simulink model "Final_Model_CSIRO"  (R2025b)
settings: Solver=ode23tb  StartTime=0.0  StopTime=50  RelTol=1e-3
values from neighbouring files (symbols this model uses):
  C_4 = 0.1670*C_b    (= 1.00487241952e-06)    [VSM_CSIRO.m]    (also in VSM.m)
  C_6 = 0.2835*C_b    (= 1.70587623314e-06)    [VSM_CSIRO.m]    (also in VSM.m)
  C_8 = 0.2275*C_b    (= 1.36891302659e-06)    [VSM_CSIRO.m]    (also in VSM.m)
  C_dc = 0.008*(n)    (= 1.6)    [VSM_CSIRO.m]    (also in VSM.m)
  C_f = n*300*10^-6    (= 0.06)    [VSM_CSIRO.m]    (also in VSM.m)
  D_p = (1/(m_p*w_b))    (= 101321.183642)    [VSM_CSIRO.m]    (also in VSM.m)
  droop_percentage = 1    [VSM_CSIRO.m]    (also in VSM.m = 5)
  i_ll = -1.15*(S_b/Vdc_n)-i_loss_dc    [VSM_CSIRO.m]    (also in VSM.m)
  i_ul = 1.15*(S_b/Vdc_n)+i_loss_dc    [VSM_CSIRO.m]    (also in VSM.m)
  J = D_p*tau_f    (= 2026.42367285)    [VSM_CSIRO.m]    (also in VSM.m)
  k_dc = eta_1/(Vdc_n*m_p)    [VSM_CSIRO.m]    (also in VSM.m)
  K_p = (1/Vdc_n)    [VSM_CSIRO.m]    (also in VSM.m)
  K_r = 1/R_dc    [VSM_CSIRO.m]    (also in VSM.m)
  Kff_i = 1    [VSM_CSIRO.m]    (also in VSM.m)
  Kff_v = 1    [VSM_CSIRO.m]    (also in VSM.m)
  Ki_i = (1/n)*1.19    (= 0.00595)    [VSM_CSIRO.m]    (also in VSM.m)
  Ki_v = (n)*1.161022    (= 232.2044)    [VSM_CSIRO.m]    (also in VSM.m)
  ki_v_ac = 4*5.2500e-04    (= 0.0021)    [VSM_CSIRO.m]    (also in VSM.m)
  Kp_i = 0.738891    [VSM_CSIRO.m]    (also in VSM.m)
  Kp_v = 0.52    [VSM_CSIRO.m]    (also in VSM.m)
  kp_v_ac = 0.001    [VSM_CSIRO.m]    (also in VSM.m)
  L1_pu = 1*0.0186/m    (= 0.000186)    [VSM_CSIRO.m]    (also in VSM.m)
  L_45 = L_lines(2)    [VSM_CSIRO.m]    (also in VSM.m)
  L_56 = L_lines(3)    [VSM_CSIRO.m]    (also in VSM.m)
  L_67 = L_lines(5)    [VSM_CSIRO.m]    (also in VSM.m)
  L_78 = L_lines(6)    [VSM_CSIRO.m]    (also in VSM.m)
  L_89 = L_lines(8)    [VSM_CSIRO.m]    (also in VSM.m)
  L_94 = L_lines(9)    [VSM_CSIRO.m]    (also in VSM.m)
  L_f = (1/n)*200*10^-6    (= 1e-06)    [VSM_CSIRO.m]    (also in VSM.m)
  n = 200    [VSM_CSIRO.m]    (also in VSM.m)
  pl = S_b*ps    (= 75000000)    [VSM_CSIRO.m]    (also in VSM.m)
  ps = base/3    (= 0.75)    [VSM_CSIRO.m]    (also in VSM.m)
  R1_pu = 1*0.00734/m    (= 7.34e-05)    [VSM_CSIRO.m]    (also in VSM.m)
  R_45 = R_lines(2)    [VSM_CSIRO.m]    (also in VSM.m)
  R_56 = R_lines(3)    [VSM_CSIRO.m]    (also in VSM.m)
  R_67 = R_lines(5)    [VSM_CSIRO.m]    (also in VSM.m)
  R_78 = R_lines(6)    [VSM_CSIRO.m]    (also in VSM.m)
  R_89 = R_lines(8)    [VSM_CSIRO.m]    (also in VSM.m)
  R_94 = R_lines(9)    [VSM_CSIRO.m]    (also in VSM.m)
  R_dc = (Vdc_n/(0.05*(S_b)/Vdc_n))    [VSM_CSIRO.m]    (also in VSM.m)
  R_f = 0.001/n    (= 5e-06)    [VSM_CSIRO.m]    (also in VSM.m)
  S_b = 100*(10^6)    (= 100000000)    [VSM_CSIRO.m]    (also in VSM.m)
  S_bt = S_b    (= 100000000)    [VSM_CSIRO.m]    (also in VSM.m)
  T_en = T_load-0.5    (= 44.5)    [VSM_CSIRO.m]    (also in VSM.m = 24.5)
  t_l = 2    [VSM_CSIRO.m]
  tau_dc = 0.05    [VSM_CSIRO.m]    (also in VSM.m)
  tau_g = 5    [VSM_CSIRO.m]    (also in VSM.m)
  V1_rms = 1000    [VSM_CSIRO.m]    (also in VSM.m)
  V2_rms = 13800    [VSM_CSIRO.m]    (also in VSM.m)
  V_m = sqrt(2/3)*V1_rms    [VSM_CSIRO.m]    (also in VSM.m)
  Vdc_n = 3*V_m    [VSM_CSIRO.m]    (also in VSM.m)
  w_b = 2*pi*f_b    (= 314.159265359)    [VSM_CSIRO.m]    (also in VSM.m)
  w_f = 2*pi*5    (= 31.4159265359)    [VSM_CSIRO.m]    (also in VSM.m)
undefined symbols (not defined in the file or in its folder): D1, Delta, DiscIntNeverNeededParam, i_dc
libraries: spsSeriesRLCBranchLib x142, spsThreePhaseVIMeasurementLib x69, slpidlib x44, spsabctodq0Lib x44, spsVoltageMeasurementLib x28, spsGroundLib x23, spsThreePhaseBreakerLib x23, spsThreePhaseParallelRLCLoadLib x21, spsdq0toabcLib x16, spsUniversalBridgeLib x16, spsPowerPositiveSequenceLib x14, spsDCVoltageSourceLib x14
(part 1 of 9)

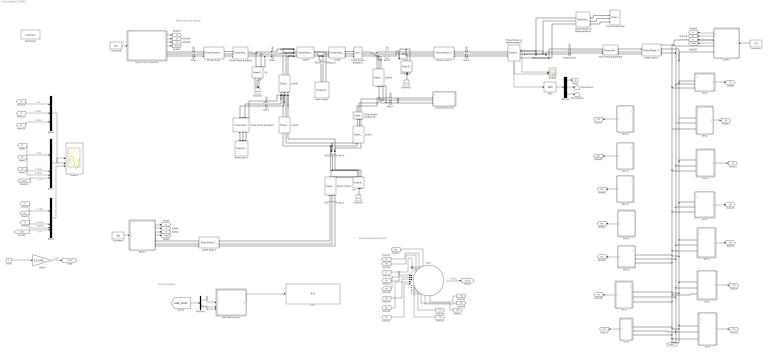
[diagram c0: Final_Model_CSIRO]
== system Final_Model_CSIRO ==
  note: Summation Block for GFLs
  note: IEEE 9-bus Test System
  note: SCR Calculation
  " " : spsThreePhaseVIMeasurementLib/Three-Phase V-I Measurement  VoltageMeasurement=no  SetLabelV=on  LabelV=Vabc_8  Vpu=on  VpuLL=off  CurrentMeasurement=no  SetLabelI=on  LabelI=Iabc_8  Ipu=on  Pbase=S_b  Vbase=V_b  OutputType=Complex  PhasorSimulation=off  PSBequivalent=0
  Base Load 5 : spsThreePhaseParallelRLCLoadLib/Three-Phase Parallel RLC Load  LConnTagsString=A|B|C  Configuration=Y (grounded)  NominalVoltage=230e3  Vabc=[1e3 1e3 1e3]  Vabcp=[1e3 1e3 1e3]  NominalFrequency=50  UnbalancedPower=off  ActivePower=pl  InductivePower=0  CapacitivePower=0  Pabc=[10e3 9e3 11e3]  QLabc=[100 90 110]  QCabc=[100 90 110]  Pabcp=[10e3 9e3 11e3]  QLabcp=[100 90 110]  QCabcp=[100 90 110]  Measurements=None  LoadType=constant Z
  "Base Load 9 " : spsThreePhaseParallelRLCLoadLib/Three-Phase Parallel RLC Load  LConnTagsString=A|B|C  Configuration=Y (grounded)  NominalVoltage=230e3  Vabc=[1e3 1e3 1e3]  Vabcp=[1e3 1e3 1e3]  NominalFrequency=50  UnbalancedPower=off  ActivePower=pl  InductivePower=0  CapacitivePower=0  Pabc=[10e3 9e3 11e3]  QLabc=[100 90 110]  QCabc=[100 90 110]  Pabcp=[10e3 9e3 11e3]  QLabcp=[100 90 110]  QCabcp=[100 90 110]  Measurements=None  LoadType=constant Z
  Bus 2 : spsThreePhaseVIMeasurementLib/Three-Phase V-I Measurement  VoltageMeasurement=no  SetLabelV=on  LabelV=Vabc_8  Vpu=on  VpuLL=off  CurrentMeasurement=no  SetLabelI=on  LabelI=Iabc_8  Ipu=on  Pbase=S_b  Vbase=V_b  OutputType=Complex  PhasorSimulation=off  PSBequivalent=0
  Bus 3 : spsThreePhaseVIMeasurementLib/Three-Phase V-I Measurement  VoltageMeasurement=no  SetLabelV=off  LabelV=Vabc_6  Vpu=off  VpuLL=off  CurrentMeasurement=no  SetLabelI=off  LabelI=Iabc_6  Ipu=off  Pbase=S_b  Vbase=V_b  OutputType=Complex  PhasorSimulation=off  PSBequivalent=0
  Bus 5 : spsThreePhaseVIMeasurementLib/Three-Phase V-I Measurement  VoltageMeasurement=no  SetLabelV=on  LabelV=Vabc_5  Vpu=on  VpuLL=off  CurrentMeasurement=no  SetLabelI=on  LabelI=Iabc_5  Ipu=on  Pbase=S_b  Vbase=V_b  OutputType=Complex  PhasorSimulation=off  PSBequivalent=0
  Bus 6 : spsThreePhaseVIMeasurementLib/Three-Phase V-I Measurement  VoltageMeasurement=no  SetLabelV=off  LabelV=Vabc_6  Vpu=off  VpuLL=off  CurrentMeasurement=no  SetLabelI=off  LabelI=Iabc_6  Ipu=off  Pbase=S_b  Vbase=V_b  OutputType=Complex  PhasorSimulation=off  PSBequivalent=0
  Bus 7 : spsThreePhaseVIMeasurementLib/Three-Phase V-I Measurement  VoltageMeasurement=no  SetLabelV=on  LabelV=Vabc_5  Vpu=on  VpuLL=off  CurrentMeasurement=no  SetLabelI=on  LabelI=Iabc_5  Ipu=on  Pbase=S_b  Vbase=V_b  OutputType=Complex  PhasorSimulation=off  PSBequivalent=0
  Bus 8 : spsThreePhaseVIMeasurementLib/Three-Phase V-I Measurement  VoltageMeasurement=no  SetLabelV=on  LabelV=Vabc_8  Vpu=on  VpuLL=off  CurrentMeasurement=no  SetLabelI=on  LabelI=Iabc_8  Ipu=on  Pbase=S_b  Vbase=V_b  OutputType=Complex  PhasorSimulation=off  PSBequivalent=0
  Bus 9 : spsThreePhaseVIMeasurementLib/Three-Phase V-I Measurement  VoltageMeasurement=no  SetLabelV=on  LabelV=Vabc_9  Vpu=on  VpuLL=off  CurrentMeasurement=no  SetLabelI=on  LabelI=Iabc_9  Ipu=on  Pbase=S_b  Vbase=V_b  OutputType=Complex  PhasorSimulation=off  PSBequivalent=0
  Bus1 : spsThreePhaseVIMeasurementLib/Three-Phase V-I Measurement  VoltageMeasurement=no  SetLabelV=on  LabelV=Vabc_1  Vpu=on  VpuLL=off  CurrentMeasurement=no  SetLabelI=on  LabelI=Iabc_1  Ipu=on  Pbase=S_b  Vbase=V_b  OutputType=Complex  PhasorSimulation=off  PSBequivalent=0
  Bus4 : spsThreePhaseVIMeasurementLib/Three-Phase V-I Measurement  VoltageMeasurement=no  SetLabelV=on  LabelV=Vabc_4  Vpu=on  VpuLL=off  CurrentMeasurement=no  SetLabelI=on  LabelI=Iabc_4  Ipu=on  Pbase=S_b  Vbase=V_b  OutputType=Complex  PhasorSimulation=off  PSBequivalent=0
  C4 : spsThreePhaseParallelRLCBranchLib/Three-Phase Parallel RLC Branch  LConnTagsString=A|B|C  RConnTagsString=A|B|C  BranchType=C  Resistance=1  Inductance=1e-3  Capacitance=C_4  Measurements=None
  C6 : spsThreePhaseParallelRLCBranchLib/Three-Phase Parallel RLC Branch  LConnTagsString=A|B|C  RConnTagsString=A|B|C  BranchType=C  Resistance=1  Inductance=1e-3  Capacitance=C_6  Measurements=None
  C8 : spsThreePhaseParallelRLCBranchLib/Three-Phase Parallel RLC Branch  LConnTagsString=A|B|C  RConnTagsString=A|B|C  BranchType=C  Resistance=1  Inductance=1e-3  Capacitance=C_8  Measurements=None
  Constant1 : Constant  Value=ps
  Constant3 : Constant  Value=0.1
  Constant8 : Constant  Value=ps
  Demux : Demux  Outputs=3
  Demux1 : Demux  Outputs=3
  Dummy Bus : spsThreePhaseVIMeasurementLib/Three-Phase V-I Measurement  VoltageMeasurement=no  SetLabelV=on  LabelV=Vabc_8  Vpu=on  VpuLL=off  CurrentMeasurement=no  SetLabelI=on  LabelI=Iabc_8  Ipu=on  Pbase=S_b  Vbase=V_b  OutputType=Complex  PhasorSimulation=off  PSBequivalent=0
  From : From
  GFL1 : Subsystem
  GFL10 : Subsystem
  GFL11 : Subsystem
  GFL12 : Subsystem
  GFL13 : Subsystem
  GFL14 : Subsystem
  GFL2 : Subsystem
  GFL3 : Subsystem
  GFL4 : Subsystem
  GFL5 : Subsystem
  GFL6 : Subsystem
  GFL7 : Subsystem
  GFL8 : Subsystem
  GFL9 : Subsystem
  GFM 1 : Subsystem
  GFM 2 : Subsystem
  Gain4 : Gain  Gain=1/(13.8e3)
  Goto7 : Goto
  Ground1 : spsGroundLib/Ground  LConnTagsString=a
  Ground2 : spsGroundLib/Ground  LConnTagsString=a
  Ground3 : spsGroundLib/Ground  LConnTagsString=a
  Incremental Load : Subsystem
  LV/MV Trafo 1 : spsThreePhaseTransformerTwoWindingsLib/Three-Phase Transformer (Two Windings)  Winding1Connection=Yg  Winding2Connection=Yg  CoreType=Three single-phase transformers  SetSaturation=off  Hysteresis=off  DataFile='hysteresis'  SetInitialFlux=off  Measurements=None  UNITS=pu  NominalPower=[S_bt 50 ]  Winding1="[ V1_rms R1_pu  L1_pu]"  Winding2=[ V2_rms R1_pu L1_pu]  Rm=Rm_pu  Lm=Lm_pu  L0=0.5  Saturation="[ 0,0  ;  0.005,1.2  ;  1.0,1.4 ]"  InitialFluxes=[ 0.8 , -0.8 , 0.7 ]  BreakLoop=off  DiscreteSolver=Trapezoidal iterative  DataType=off  TransfoNumber=0
  LV/MV Trafo 2 : spsThreePhaseTransformerTwoWindingsLib/Three-Phase Transformer (Two Windings)  Winding1Connection=Yg  Winding2Connection=Yg  CoreType=Three single-phase transformers  SetSaturation=off  Hysteresis=off  DataFile='hysteresis'  SetInitialFlux=off  Measurements=None  UNITS=pu  NominalPower=[ S_bt 50 ]  Winding1="[ V1_rms R1_pu  L1_pu]"  Winding2=[ V2_rms R1_pu L1_pu]  Rm=Rm_pu  Lm=Lm_pu  L0=0.5  Saturation="[ 0,0  ;  0.005,1.2  ;  1.0,1.4 ]"  InitialFluxes=[ 0.8 , -0.8 , 0.7 ]  BreakLoop=off  DiscreteSolver=Trapezoidal iterative  DataType=off  TransfoNumber=0
  Line45 : spsThreePhaseSeriesRLCBranchLib/Three-Phase Series RLC Branch  LConnTagsString=A|B|C  RConnTagsString=A|B|C  BranchType=RL  Resistance=R_45  Inductance=L_45  Capacitance=0  Measurements=None
  Line56 : spsThreePhaseSeriesRLCBranchLib/Three-Phase Series RLC Branch  LConnTagsString=A|B|C  RConnTagsString=A|B|C  BranchType=RL  Resistance=R_56  Inductance=L_56  Capacitance=0  Measurements=None
  Line67 : spsThreePhaseSeriesRLCBranchLib/Three-Phase Series RLC Branch  LConnTagsString=A|B|C  RConnTagsString=A|B|C  BranchType=RL  Resistance=R_67  Inductance=L_67  Capacitance=0  Measurements=None
  Line78 : spsThreePhaseSeriesRLCBranchLib/Three-Phase Series RLC Branch  LConnTagsString=A|B|C  RConnTagsString=A|B|C  BranchType=RL  Resistance=R_78  Inductance=L_78  Capacitance=0  Measurements=None
  Line89 : spsThreePhaseSeriesRLCBranchLib/Three-Phase Series RLC Branch  LConnTagsString=A|B|C  RConnTagsString=A|B|C  BranchType=RL  Resistance=R_89  Inductance=L_89  Capacitance=0  Measurements=None
  Line94 : spsThreePhaseSeriesRLCBranchLib/Three-Phase Series RLC Branch  LConnTagsString=A|B|C  RConnTagsString=A|B|C  BranchType=RL  Resistance=R_94  Inductance=L_94  Capacitance=0  Measurements=None
  MATLAB Function : MATLAB Function  TreatAsAtomicUnit=on
  "MV/HV Trafo " : spsThreePhaseTransformerTwoWindingsLib/Three-Phase Transformer (Two Windings)  Winding1Connection=Delta (D1)  Winding2Connection=Yg  CoreType=Three single-phase transformers  SetSaturation=off  Hysteresis=off  DataFile='hysteresis'  SetInitialFlux=off  Measurements=None  UNITS=pu  NominalPower=[ 210e6 50 ]  Winding1="[V2_rms 0.0027  0.08]"  Winding2=[230e3 0.0027 0.08]  Rm=500  Lm=500  L0=0.5  Saturation="[ 0,0  ;  0.005,1.2  ;  1.0,1.4 ]"  InitialFluxes=[ 0.8 , -0.8 , 0.7 ]  BreakLoop=off  DiscreteSolver=Trapezoidal iterative  DataType=off  TransfoNumber=0
  "MV/HV Trafo 1 " : spsThreePhaseTransformerTwoWindingsLib/Three-Phase Transformer (Two Windings)  Winding1Connection=Yg  Winding2Connection=Yg  CoreType=Three single-phase transformers  SetSaturation=off  Hysteresis=off  DataFile='hysteresis'  SetInitialFlux=off  Measurements=None  UNITS=pu  NominalPower=[ 210e6 50 ]  Winding1=[V2_rms 0.0027 0.08]  Winding2=[ 230e3 0.0027 0.08]  Rm=500  Lm=500  L0=0.5  Saturation="[ 0,0  ;  0.005,1.2  ;  1.0,1.4 ]"  InitialFluxes=[ 0.8 , -0.8 , 0.7 ]  BreakLoop=off  DiscreteSolver=Trapezoidal iterative  DataType=off  TransfoNumber=0
  "MV/HV Trafo 2 " : spsThreePhaseTransformerTwoWindingsLib/Three-Phase Transformer (Two Windings)  Winding1Connection=Yg  Winding2Connection=Yg  CoreType=Three single-phase transformers  SetSaturation=off  Hysteresis=off  DataFile='hysteresis'  SetInitialFlux=off  Measurements=None  UNITS=pu  NominalPower=[ 210e6 50 ]  Winding1=[V2_rms 0.0027 0.08]  Winding2=[230e3 0.0027 0.08]  Rm=500  Lm=500  L0=0.5  Saturation="[ 0,0  ;  0.005,1.2  ;  1.0,1.4 ]"  InitialFluxes=[ 0.8 , -0.8 , 0.7 ]  BreakLoop=off  DiscreteSolver=Trapezoidal iterative  DataType=off  TransfoNumber=0
  Mux1 : Mux
  Mux2 : Mux
  Mux6 : Mux  Inputs=3
  Power2 : Scope  NumInputPorts=3
  RMS : spsRMSLib/RMS  TrueRMS=on  Freq=50  RMSInit=120  Ts=0
  SCR : Display
  Scope1 : Scope  NumInputPorts=2
  Sum : Sum  Inputs=|++++++++++++++
  Synchronous Machine : Subsystem
  Terminator1 : Terminator
  Terminator2 : Terminator
  Three-Phase V-I Measurement1 : spsThreePhaseVIMeasurementLib/Three-Phase V-I Measurement  VoltageMeasurement=phase-to-phase  SetLabelV=off  LabelV=Vabc  Vpu=off  VpuLL=off  CurrentMeasurement=yes  SetLabelI=off  LabelI=Iabc  Ipu=off  Pbase=100e6  Vbase=500e3  OutputType=Complex  PhasorSimulation=off  PSBequivalent=0
  Three-Phase V-I Measurement3 : spsThreePhaseVIMeasurementLib/Three-Phase V-I Measurement  VoltageMeasurement=phase-to-phase  SetLabelV=on  LabelV=Vabc_Fault  Vpu=off  VpuLL=off  CurrentMeasurement=yes  SetLabelI=on  LabelI=Iabc_Fault  Ipu=off  Pbase=100e6  Vbase=500e3  OutputType=Complex  PhasorSimulation=off  PSBequivalent=0
  Three-Phase Breaker1 : spsThreePhaseBreakerLib/Three-Phase Breaker  InitialState=closed  SwitchA=on  SwitchB=on  SwitchC=on  SwitchTimes=50  External=off  BreakerResistance=1  SnubberResistance=1e6  SnubberCapacitance=inf  Measurements=None
  Three-Phase Breaker10 : spsThreePhaseBreakerLib/Three-Phase Breaker  InitialState=open  SwitchA=on  SwitchB=on  SwitchC=on  SwitchTimes=[0 0.5 40]  External=off  BreakerResistance=0.01  SnubberResistance=1e6  SnubberCapacitance=inf  Measurements=None
  Three-Phase Breaker5 : spsThreePhaseBreakerLib/Three-Phase Breaker  InitialState=open  SwitchA=on  SwitchB=on  SwitchC=on  SwitchTimes=1  External=off  BreakerResistance=0.01  SnubberResistance=1e6  SnubberCapacitance=inf  Measurements=None
  Three-Phase Breaker6 : spsThreePhaseBreakerLib/Three-Phase Breaker  InitialState=open  SwitchA=on  SwitchB=on  SwitchC=on  SwitchTimes=10  External=off  BreakerResistance=0.01  SnubberResistance=1e6  SnubberCapacitance=inf  Measurements=None
  Three-Phase Breaker9 : spsThreePhaseBreakerLib/Three-Phase Breaker  InitialState=open  SwitchA=on  SwitchB=on  SwitchC=on  SwitchTimes=[0 0.5 35]  External=off  BreakerResistance=0.01  SnubberResistance=1e6  SnubberCapacitance=inf  Measurements=None
  Three-Phase Fault : spsThreePhaseFaultLib/Three-Phase Fault  InitialStates=0  FaultA=on  FaultB=on  FaultC=on  GroundFault=on  SwitchTimes=[0.1 0.2]  External=off  SwitchStatus=NaN  FaultResistance=0.001  GroundResistance=0.01  SnubberResistance=1e6  SnubberCapacitance=inf  Measurements=Fault voltages and currents
  powergui2 : sps_lib/powergui  Priority=1  SimulationMode=Discrete  SampleTime=1e-4  frequency=50  Iterations=50  frequencyindice=0  Pbase=100e6  ErrMax=0.0001  UnitsV=kV  UnitsW=MW  buscounter=0  FunctionMessages=off  echomessages=off  EnableUseOfTLC=off  CurrentSourceSwitches=off  DisableSnubberDevices=off  DisableRonSwitches=off  DisableVfSwitches=off  DisplayEquations=off  AutomaticDiscreteSolvers=off  SolverType=Tustin/Backward Euler (TBE)  Interpol=off  ExternalGateDelay=off  methode=off  Ts=100  x0status=blocks  SPID=off  SwTol=0  HookPort=off  NonlinearTolerance=1e-4  nMaxIteration=100  ContinueOnMaxIteration=off  RestoreLinks=warning  ResistiveCurrentMeasurement=off  Frange=[0:2:500]  Ylog=off  Xlog=on  ShowGrid=off  save=off  variable=ZData  structure=0  ZoomFFT=off  StartTime=0.0  cycles=1  DisplayStyle=1  fundamental=60  FreqAxis=off  MaxFrequency=1000  frequencyindicesteady=1  RmsSteady=1  display=off
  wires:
  [f1] -> Mux6/1  "f_SM"
  GFM 1/2(V) -> [V2]
  GFM 2/2(V) -> [V3]
  GFM 2/1(f) -> [f3]
  [P3] -> Mux1/3  "P_GFM2"
  Constant1/1 -> GFM 2/1(Pset)
  [P2] -> Mux1/2  "P_GFM1"
  GFM 2/3(P) -> [P3]
  GFM 1/4(Theta) -> [Theta2]
  [V1] -> Mux2/1  "V_SM"
  Synchronous Machine/1(f) -> [f1]
  GFM 1/3(P) -> [P2]
  [f3] -> Mux6/3  "f_GFM2"
  [P1] -> Mux1/1  "P_SM"
  [V3] -> Mux2/3  "V_GFM2"
  Constant8/1 -> Synchronous Machine/1(Pset)
  Mux6/1 -> Power2/1
  GFM 1/1(f) -> [f2]
  [V2] -> Mux2/2  "V_GFM1"
  Mux1/1 -> Power2/2
  Synchronous Machine/3(P) -> [P1]
  Synchronous Machine/4(Theta) -> [Theta1]
  GFM 2/4(Theta) -> [Theta3]
  Synchronous Machine/2(V) -> [V1]
  Mux2/1 -> Power2/3
  [f2] -> Mux6/2  "f_GFM1"
  Three-Phase V-I Measurement1/2 -> Scope1/1
  Three-Phase V-I Measurement1/1 -> RMS/1, Scope1/2
  [V_PCC] -> Mux2/4  "V_PCC"
  [Iabc_Fault] -> Demux1/1
  Demux1/1 -> MATLAB Function/1(Ia)
  Demux1/3 -> MATLAB Function/3(Ic)
  MATLAB Function/1(SCR) -> SCR/1
  Demux1/2 -> MATLAB Function/2(Ib)
  RMS/1 -> Demux/1
  Demux/3 -> Terminator2/1
  Demux/2 -> Terminator1/1
  Demux/1 -> Goto7/1
  From/1 -> Gain4/1
  Gain4/1 -> [V_PCC]  "V_PCC"
  GFL1/1(Out1) -> [P5]
  GFL2/1(Out1) -> [P6]
  GFL3/1(Out1) -> [P7]
  GFL4/1(Out1) -> [P8]
  GFL5/1(Out1) -> [P9]
  GFL6/1(Out1) -> [P10]
  GFL7/1(Out1) -> [P11]
  [P15] -> Sum/1
  [P5] -> Sum/2
  [P6] -> Sum/3
  [P7] -> Sum/4
  [P8] -> Sum/5
  [P9] -> Sum/6
  [P10] -> Sum/7
  [P11] -> Sum/8
  Sum/1 -> [P_GFLs]  "P_GFLs"
  [P_GFLs] -> Mux1/4  "P_GFL"
  GFL8/1(Out1) -> [P12]
  [P12] -> Sum/9
  GFL10/1(Out1) -> [P13]
  [P13] -> Sum/10
  GFL9/1(Out1) -> [P14]
  [P14] -> Sum/11
  GFL11/1(Out1) -> [P15]
  GFL12/1(Out1) -> [P16]
  Constant3/1 -> GFM 1/1(Pset)
  GFL13/1(Out1) -> [P17]
  GFL14/1(Out1) -> [P18]
  [P16] -> Sum/12
  [P17] -> Sum/13
  [P18] -> Sum/14
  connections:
  Bus4/RConn2 -- Three-Phase Breaker1/RConn2 -- C4/LConn2
  "MV/HV Trafo 2 "/RConn3 -- C6/LConn3 -- Bus 6/RConn3
  Bus 8/LConn2 -- C8/LConn2 -- "MV/HV Trafo 1 "/RConn2
  C6/RConn2 -- Ground3/LConn1 -- C6/RConn1 -- C6/RConn3
  Bus 7/RConn2 -- Three-Phase Breaker10/LConn2 -- Line78/RConn2
  C4/LConn1 -- Bus4/RConn1 -- Three-Phase Breaker1/RConn1
  Line67/RConn1 -- Line56/RConn1 -- Bus 6/LConn1
  Line94/RConn3 -- Bus 9/RConn1 -- Line89/LConn3
  Bus 8/LConn3 -- C8/LConn3 -- "MV/HV Trafo 1 "/RConn3
  Bus 7/RConn3 -- Three-Phase Breaker10/LConn3 -- Line78/RConn3
  Line94/LConn1 -- Bus4/LConn1 -- Line45/LConn1
  Line45/RConn2 -- Line56/LConn2 -- Bus 5/LConn2
  Line94/LConn2 -- Bus4/LConn2 -- Line45/LConn2
  Line94/LConn3 -- Bus4/LConn3 -- Line45/LConn3
  C8/RConn2 -- C8/RConn3 -- C8/RConn1 -- Ground2/LConn1
  Line45/RConn1 -- Line56/LConn1 -- Bus 5/LConn1
  C6/LConn1 -- "MV/HV Trafo 2 "/RConn1 -- Bus 6/RConn1
  Line45/RConn3 -- Line56/LConn3 -- Bus 5/LConn3
  Bus 9/RConn2 -- Line94/RConn2 -- Line89/LConn2
  Ground1/LConn1 -- C4/RConn2 -- C4/RConn3 -- C4/RConn1
  Bus 7/RConn1 -- Three-Phase Breaker10/LConn1 -- Line78/RConn1
  Bus 6/LConn2 -- Line67/RConn2 -- Line56/RConn2
  Bus 6/LConn3 -- Line56/RConn3 -- Line67/RConn3
  Line94/RConn1 -- Bus 9/RConn3 -- Line89/LConn1
  Bus 8/LConn1 -- C8/LConn1 -- "MV/HV Trafo 1 "/RConn1
  C6/LConn2 -- "MV/HV Trafo 2 "/RConn2 -- Bus 6/RConn2
  Bus4/RConn3 -- Three-Phase Breaker1/RConn3 -- C4/LConn3
  Bus 2/RConn1 -- "MV/HV Trafo 1 "/LConn3
  Bus 2/RConn2 -- "MV/HV Trafo 1 "/LConn2
  GFM 2/RConn3 -- LV/MV Trafo 2/LConn3
  GFM 2/RConn2 -- LV/MV Trafo 2/LConn2
  GFM 2/RConn1 -- LV/MV Trafo 2/LConn1
  Bus1/LConn3 -- "MV/HV Trafo "/LConn3
  Bus 2/RConn3 -- "MV/HV Trafo 1 "/LConn1
  "Base Load 9 "/LConn1 -- Bus 9/LConn3
  "Base Load 9 "/LConn3 -- Bus 9/LConn1
  Bus1/LConn2 -- "MV/HV Trafo "/LConn2
  Bus 3/LConn1 -- "MV/HV Trafo 2 "/LConn1
  "Base Load 9 "/LConn2 -- Bus 9/LConn2
  Bus 3/LConn3 -- "MV/HV Trafo 2 "/LConn3
  Bus1/LConn1 -- "MV/HV Trafo "/LConn1
  Bus 3/LConn2 -- "MV/HV Trafo 2 "/LConn2
  "MV/HV Trafo "/RConn1 -- Three-Phase Breaker1/LConn1
  "MV/HV Trafo "/RConn2 -- Three-Phase Breaker1/LConn2
  "MV/HV Trafo "/RConn3 -- Three-Phase Breaker1/LConn3
  GFL2/LConn3 -- GFL3/LConn3 -- GFL4/LConn3 -- GFL5/LConn3 -- GFL10/LConn3 -- GFL6/LConn3 -- GFL9/LConn3 -- GFL8/LConn3 -- GFL7/LConn3 -- " "/LConn3 -- LV/MV Trafo 1/LConn3 -- GFM 1/RConn1 -- GFL1/LConn3
  Bus 3/RConn1 -- LV/MV Trafo 2/RConn1
  Bus 3/RConn2 -- LV/MV Trafo 2/RConn2
  Bus 3/RConn3 -- LV/MV Trafo 2/RConn3
  Synchronous Machine/RConn2 -- Bus1/RConn2
  Synchronous Machine/RConn3 -- Bus1/RConn3
  Synchronous Machine/RConn1 -- Bus1/RConn1
  Incremental Load/LConn1 -- Bus 7/LConn3
  Three-Phase Breaker6/RConn2 -- Base Load 5/LConn2
  Three-Phase Breaker6/RConn3 -- Base Load 5/LConn1
  Three-Phase Breaker6/RConn1 -- Base Load 5/LConn3
  Bus 5/RConn1 -- Three-Phase Breaker6/LConn1
  Bus 5/RConn2 -- Three-Phase Breaker6/LConn2
  Bus 5/RConn3 -- Three-Phase Breaker6/LConn3
  Three-Phase V-I Measurement1/LConn1 -- Bus 2/LConn3
  Three-Phase V-I Measurement1/LConn2 -- Bus 2/LConn2
  Three-Phase V-I Measurement1/LConn3 -- Bus 2/LConn1
  Three-Phase Breaker5/LConn1 -- LV/MV Trafo 1/RConn1
  Three-Phase Breaker5/LConn2 -- LV/MV Trafo 1/RConn2
  Three-Phase Breaker5/LConn3 -- LV/MV Trafo 1/RConn3
  Three-Phase V-I Measurement1/RConn3 -- Three-Phase V-I Measurement3/RConn3 -- Dummy Bus/RConn1
  Three-Phase V-I Measurement1/RConn2 -- Three-Phase V-I Measurement3/RConn2 -- Dummy Bus/RConn2
  Three-Phase V-I Measurement1/RConn1 -- Three-Phase V-I Measurement3/RConn1 -- Dummy Bus/RConn3
  Three-Phase V-I Measurement3/LConn1 -- Three-Phase Fault/LConn1
  Three-Phase V-I Measurement3/LConn2 -- Three-Phase Fault/LConn2
  Three-Phase V-I Measurement3/LConn3 -- Three-Phase Fault/LConn3
  Dummy Bus/LConn2 -- Three-Phase Breaker5/RConn2
  Dummy Bus/LConn3 -- Three-Phase Breaker5/RConn1
  Dummy Bus/LConn1 -- Three-Phase Breaker5/RConn3
  Line89/RConn1 -- Three-Phase Breaker9/RConn1
  Three-Phase Breaker9/RConn3 -- Line89/RConn3
  Three-Phase Breaker9/RConn2 -- Line89/RConn2
  Three-Phase Breaker10/RConn1 -- Line67/LConn1
  Three-Phase Breaker10/RConn2 -- Line67/LConn2
  Three-Phase Breaker10/RConn3 -- Line67/LConn3
  Line78/LConn1 -- Three-Phase Breaker9/LConn1 -- Bus 8/RConn1
  Line78/LConn2 -- Three-Phase Breaker9/LConn2 -- Bus 8/RConn2
  Line78/LConn3 -- Three-Phase Breaker9/LConn3 -- Bus 8/RConn3
  Incremental Load/LConn3 -- Bus 7/LConn1
  GFL2/LConn1 -- GFL3/LConn1 -- GFL4/LConn1 -- GFL5/LConn1 -- GFL10/LConn1 -- GFL6/LConn1 -- GFL9/LConn1 -- GFL7/LConn1 -- GFL8/LConn1 -- " "/LConn1 -- GFM 1/RConn3 -- LV/MV Trafo 1/LConn1 -- GFL1/LConn1
  GFL2/LConn2 -- GFL3/LConn2 -- GFL4/LConn2 -- GFL5/LConn2 -- GFL10/LConn2 -- GFL6/LConn2 -- GFL9/LConn2 -- GFL8/LConn2 -- GFL7/LConn2 -- " "/LConn2 -- GFL1/LConn2 -- LV/MV Trafo 1/LConn2 -- GFM 1/RConn2
  Incremental Load/LConn2 -- Bus 7/LConn2

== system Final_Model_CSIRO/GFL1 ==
  B1 : spsThreePhaseVIMeasurementLib/Three-Phase V-I Measurement  VoltageMeasurement=phase-to-ground  SetLabelV=on  LabelV=Vabc_B1_2  Vpu=off  VpuLL=off  CurrentMeasurement=yes  SetLabelI=on  LabelI=Iabc_B1_2  Ipu=off  Pbase=100e6  Vbase=500e3  OutputType=Complex  PhasorSimulation=off  PSBequivalent=0
  B3 : spsThreePhaseVIMeasurementLib/Three-Phase V-I Measurement  VoltageMeasurement=phase-to-ground  SetLabelV=on  LabelV=Vabc_B3_2  Vpu=off  VpuLL=off  CurrentMeasurement=yes  SetLabelI=on  LabelI=Iabc_B3_2  Ipu=off  Pbase=100e6  Vbase=500e3  OutputType=Complex  PhasorSimulation=off  PSBequivalent=0
  B4 : spsThreePhaseVIMeasurementLib/Three-Phase V-I Measurement  VoltageMeasurement=phase-to-ground  SetLabelV=on  LabelV=Vabc_B4_2  Vpu=off  VpuLL=off  CurrentMeasurement=yes  SetLabelI=on  LabelI=Iabc_B4_2  Ipu=off  Pbase=100e6  Vbase=500e3  OutputType=Complex  PhasorSimulation=off  PSBequivalent=0
  Constant1 : Constant  Value=0  SampleTime=-1
  Gain2 : Gain  Gain=1e-8
  Inverter Control : Subsystem
  LCL Filter : Subsystem
  Power (Positive-Sequence) : spsPowerPositiveSequenceLib/Power (Positive-Sequence)  Freq=50  Vinit=[0, 0]  Iinit=[0, 0]  Ts=0
  Scope : Scope  NumInputPorts=4
  Scope1 : Scope
  Step : Step  Time=12  After=8200  SampleTime=0
  Universal Bridge : spsUniversalBridgeLib/Universal Bridge  Arms=3  SnubberResistance=1e5  SnubberCapacitance=inf  Device=Average-model based VSC  Ron=1e-3  Lon=0  ForwardVoltages="[  0  0  ]"  ForwardVoltage=0  GTOparameters=[ 10e-6 , 20e-6 ]  IGBTparameters=[ 1e-6 , 2e-6 ]  Measurements=None  Measurements_2=None  converterType=Rectifier
  Vdc : spsDCVoltageSourceLib/DC Voltage Source  Amplitude=1800  Measurements=None
  Voltage Measurement1 : spsVoltageMeasurementLib/Voltage Measurement  PhasorSimulation=off  OutputType=Complex  PSBequivalent=0
  Connection Port : PMIOPort  Side=Left
  Connection Port1 : PMIOPort  Port=2  Side=Left
  Connection Port2 : PMIOPort  Port=3  Side=Left
  Out1 : Outport
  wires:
  [Vabc_B1_2] -> Scope/3  "Inverter Voltage"
  [Iabc_B1_2] -> Scope/4  "Inverter Current"
  Voltage Measurement1/1 -> Scope1/1
  [Iabc_B3_2] -> Power (Positive-Sequence)/2, Scope/2  "PCC Current"
  Inverter Control/1(Pulses) -> Universal Bridge/1
  [Vabc_B3_2] -> Inverter Control/1(Vabc_B3)
  [Iabc_B3_2] -> Inverter Control/2(Iabc_B3)
  [Vabc_B3_2] -> Scope/1, Power (Positive-Sequence)/1  "PCC Voltage"
  Power (Positive-Sequence)/1 -> Gain2/1
  Gain2/1 -> Out1/1
  Constant1/1 -> Inverter Control/4(Iqref)
  Step/1 -> Inverter Control/3(Idref)
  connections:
  Universal Bridge/RConn1 -- Vdc/RConn1
  Universal Bridge/RConn2 -- Vdc/LConn1
  B1/LConn2 -- Voltage Measurement1/LConn2 -- Universal Bridge/LConn2
  Universal Bridge/LConn1 -- Voltage Measurement1/LConn1 -- B1/LConn1
  B3/LConn3 -- LCL Filter/RConn3
  B3/RConn3 -- B4/LConn3
  B3/RConn1 -- B4/LConn1
  Connection Port2/RConn1 -- B4/RConn3
  B3/LConn2 -- LCL Filter/RConn2
  Universal Bridge/LConn3 -- B1/LConn3
  B3/RConn2 -- B4/LConn2
  B3/LConn1 -- LCL Filter/RConn1
  B1/RConn1 -- LCL Filter/LConn1
  B1/RConn2 -- LCL Filter/LConn2
  B1/RConn3 -- LCL Filter/LConn3
  B4/RConn1 -- Connection Port/RConn1
  B4/RConn2 -- Connection Port1/RConn1

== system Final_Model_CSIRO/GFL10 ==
  B1 : spsThreePhaseVIMeasurementLib/Three-Phase V-I Measurement  VoltageMeasurement=phase-to-ground  SetLabelV=on  LabelV=Vabc_B1_10  Vpu=off  VpuLL=off  CurrentMeasurement=yes  SetLabelI=on  LabelI=Iabc_B1_10  Ipu=off  Pbase=100e6  Vbase=500e3  OutputType=Complex  PhasorSimulation=off  PSBequivalent=0
  B3 : spsThreePhaseVIMeasurementLib/Three-Phase V-I Measurement  VoltageMeasurement=phase-to-ground  SetLabelV=on  LabelV=Vabc_B3_10  Vpu=off  VpuLL=off  CurrentMeasurement=yes  SetLabelI=on  LabelI=Iabc_B3_10  Ipu=off  Pbase=100e6  Vbase=500e3  OutputType=Complex  PhasorSimulation=off  PSBequivalent=0
  B4 : spsThreePhaseVIMeasurementLib/Three-Phase V-I Measurement  VoltageMeasurement=phase-to-ground  SetLabelV=on  LabelV=Vabc_B4_10  Vpu=off  VpuLL=off  CurrentMeasurement=yes  SetLabelI=on  LabelI=Iabc_B4_10  Ipu=off  Pbase=100e6  Vbase=500e3  OutputType=Complex  PhasorSimulation=off  PSBequivalent=0
  Constant1 : Constant  Value=0  SampleTime=-1
  Gain2 : Gain  Gain=1e-8
  Inverter Control : Subsystem
  LCL Filter : Subsystem
  Power (Positive-Sequence) : spsPowerPositiveSequenceLib/Power (Positive-Sequence)  Freq=50  Vinit=[0, 0]  Iinit=[0, 0]  Ts=0
  Scope : Scope  NumInputPorts=4
  Scope1 : Scope
  Step : Step  Time=12+9*t_l  After=8200  SampleTime=0
  Universal Bridge : spsUniversalBridgeLib/Universal Bridge  Arms=3  SnubberResistance=1e5  SnubberCapacitance=inf  Device=Average-model based VSC  Ron=1e-3  Lon=0  ForwardVoltages="[  0  0  ]"  ForwardVoltage=0  GTOparameters=[ 10e-6 , 20e-6 ]  IGBTparameters=[ 1e-6 , 2e-6 ]  Measurements=None  Measurements_2=None  converterType=Rectifier
  Vdc : spsDCVoltageSourceLib/DC Voltage Source  Amplitude=1800  Measurements=None
  Voltage Measurement1 : spsVoltageMeasurementLib/Voltage Measurement  PhasorSimulation=off  OutputType=Complex  PSBequivalent=0
  Connection Port : PMIOPort  Side=Left
  Connection Port1 : PMIOPort  Port=2  Side=Left
  Connection Port2 : PMIOPort  Port=3  Side=Left
  Out1 : Outport
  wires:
  [Vabc_B1_10] -> Scope/3  "Inverter Voltage"
  [Iabc_B1_10] -> Scope/4  "Inverter Current"
  Voltage Measurement1/1 -> Scope1/1
  [Iabc_B3_10] -> Power (Positive-Sequence)/2, Scope/2  "PCC Current"
  Inverter Control/1(Pulses) -> Universal Bridge/1
  [Vabc_B3_10] -> Inverter Control/1(Vabc_B3)
  [Iabc_B3_10] -> Inverter Control/2(Iabc_B3)
  [Vabc_B3_10] -> Scope/1, Power (Positive-Sequence)/1  "PCC Voltage"
  Power (Positive-Sequence)/1 -> Gain2/1
  Gain2/1 -> Out1/1
  Constant1/1 -> Inverter Control/4(Iqref)
  Step/1 -> Inverter Control/3(Idref)
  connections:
  Universal Bridge/RConn1 -- Vdc/RConn1
  Universal Bridge/RConn2 -- Vdc/LConn1
  B1/LConn2 -- Voltage Measurement1/LConn2 -- Universal Bridge/LConn2
  Universal Bridge/LConn1 -- Voltage Measurement1/LConn1 -- B1/LConn1
  B3/LConn3 -- LCL Filter/RConn3
  B3/RConn3 -- B4/LConn3
  B3/RConn1 -- B4/LConn1
  Connection Port2/RConn1 -- B4/RConn3
  B3/LConn2 -- LCL Filter/RConn2
  Universal Bridge/LConn3 -- B1/LConn3
  B3/RConn2 -- B4/LConn2
  B3/LConn1 -- LCL Filter/RConn1
  B1/RConn1 -- LCL Filter/LConn1
  B1/RConn2 -- LCL Filter/LConn2
  B1/RConn3 -- LCL Filter/LConn3
  B4/RConn1 -- Connection Port/RConn1
  B4/RConn2 -- Connection Port1/RConn1

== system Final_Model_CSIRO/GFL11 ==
  B1 : spsThreePhaseVIMeasurementLib/Three-Phase V-I Measurement  VoltageMeasurement=phase-to-ground  SetLabelV=on  LabelV=Vabc_B1_12  Vpu=off  VpuLL=off  CurrentMeasurement=yes  SetLabelI=on  LabelI=Iabc_B1_12  Ipu=off  Pbase=100e6  Vbase=500e3  OutputType=Complex  PhasorSimulation=off  PSBequivalent=0
  B3 : spsThreePhaseVIMeasurementLib/Three-Phase V-I Measurement  VoltageMeasurement=phase-to-ground  SetLabelV=on  LabelV=Vabc_B3_12  Vpu=off  VpuLL=off  CurrentMeasurement=yes  SetLabelI=on  LabelI=Iabc_B3_12  Ipu=off  Pbase=100e6  Vbase=500e3  OutputType=Complex  PhasorSimulation=off  PSBequivalent=0
  B4 : spsThreePhaseVIMeasurementLib/Three-Phase V-I Measurement  VoltageMeasurement=phase-to-ground  SetLabelV=on  LabelV=Vabc_B4_12  Vpu=off  VpuLL=off  CurrentMeasurement=yes  SetLabelI=on  LabelI=Iabc_B4_12  Ipu=off  Pbase=100e6  Vbase=500e3  OutputType=Complex  PhasorSimulation=off  PSBequivalent=0
  Constant1 : Constant  Value=0  SampleTime=-1
  Gain2 : Gain  Gain=1e-8
  Inverter Control : Subsystem
  LCL Filter : Subsystem
  Power (Positive-Sequence) : spsPowerPositiveSequenceLib/Power (Positive-Sequence)  Freq=50  Vinit=[0, 0]  Iinit=[0, 0]  Ts=0
  Scope : Scope  NumInputPorts=4
  Scope1 : Scope
  Step : Step  Time=12+10*t_l  After=8200  SampleTime=0
  Universal Bridge : spsUniversalBridgeLib/Universal Bridge  Arms=3  SnubberResistance=1e5  SnubberCapacitance=inf  Device=Average-model based VSC  Ron=1e-3  Lon=0  ForwardVoltages="[  0  0  ]"  ForwardVoltage=0  GTOparameters=[ 10e-6 , 20e-6 ]  IGBTparameters=[ 1e-6 , 2e-6 ]  Measurements=None  Measurements_2=None  converterType=Rectifier
  Vdc : spsDCVoltageSourceLib/DC Voltage Source  Amplitude=1800  Measurements=None
  Voltage Measurement1 : spsVoltageMeasurementLib/Voltage Measurement  PhasorSimulation=off  OutputType=Complex  PSBequivalent=0
  Connection Port : PMIOPort  Side=Left
  Connection Port1 : PMIOPort  Port=2  Side=Left
  Connection Port2 : PMIOPort  Port=3  Side=Left
  Out1 : Outport
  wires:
  [Vabc_B1_12] -> Scope/3  "Inverter Voltage"
  [Iabc_B1_12] -> Scope/4  "Inverter Current"
  Voltage Measurement1/1 -> Scope1/1
  [Iabc_B3_12] -> Power (Positive-Sequence)/2, Scope/2  "PCC Current"
  Inverter Control/1(Pulses) -> Universal Bridge/1
  [Vabc_B3_12] -> Inverter Control/1(Vabc_B3)
  [Iabc_B3_12] -> Inverter Control/2(Iabc_B3)
  [Vabc_B3_12] -> Scope/1, Power (Positive-Sequence)/1  "PCC Voltage"
  Power (Positive-Sequence)/1 -> Gain2/1
  Gain2/1 -> Out1/1
  Constant1/1 -> Inverter Control/4(Iqref)
  Step/1 -> Inverter Control/3(Idref)
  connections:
  Universal Bridge/RConn1 -- Vdc/RConn1
  Universal Bridge/RConn2 -- Vdc/LConn1
  B1/LConn2 -- Voltage Measurement1/LConn2 -- Universal Bridge/LConn2
  Universal Bridge/LConn1 -- Voltage Measurement1/LConn1 -- B1/LConn1
  B3/LConn3 -- LCL Filter/RConn3
  B3/RConn3 -- B4/LConn3
  B3/RConn1 -- B4/LConn1
  Connection Port2/RConn1 -- B4/RConn3
  B3/LConn2 -- LCL Filter/RConn2
  Universal Bridge/LConn3 -- B1/LConn3
  B3/RConn2 -- B4/LConn2
  B3/LConn1 -- LCL Filter/RConn1
  B1/RConn1 -- LCL Filter/LConn1
  B1/RConn2 -- LCL Filter/LConn2
  B1/RConn3 -- LCL Filter/LConn3
  B4/RConn1 -- Connection Port/RConn1
  B4/RConn2 -- Connection Port1/RConn1

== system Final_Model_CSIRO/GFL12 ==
  B1 : spsThreePhaseVIMeasurementLib/Three-Phase V-I Measurement  VoltageMeasurement=phase-to-ground  SetLabelV=on  LabelV=Vabc_B1_13  Vpu=off  VpuLL=off  CurrentMeasurement=yes  SetLabelI=on  LabelI=Iabc_B1_13  Ipu=off  Pbase=100e6  Vbase=500e3  OutputType=Complex  PhasorSimulation=off  PSBequivalent=0
  B3 : spsThreePhaseVIMeasurementLib/Three-Phase V-I Measurement  VoltageMeasurement=phase-to-ground  SetLabelV=on  LabelV=Vabc_B3_13  Vpu=off  VpuLL=off  CurrentMeasurement=yes  SetLabelI=on  LabelI=Iabc_B3_13  Ipu=off  Pbase=100e6  Vbase=500e3  OutputType=Complex  PhasorSimulation=off  PSBequivalent=0
  B4 : spsThreePhaseVIMeasurementLib/Three-Phase V-I Measurement  VoltageMeasurement=phase-to-ground  SetLabelV=on  LabelV=Vabc_B4_13  Vpu=off  VpuLL=off  CurrentMeasurement=yes  SetLabelI=on  LabelI=Iabc_B4_13  Ipu=off  Pbase=100e6  Vbase=500e3  OutputType=Complex  PhasorSimulation=off  PSBequivalent=0
  Constant1 : Constant  Value=0  SampleTime=-1
  Gain2 : Gain  Gain=1e-8
  Inverter Control : Subsystem
  LCL Filter : Subsystem
  Power (Positive-Sequence) : spsPowerPositiveSequenceLib/Power (Positive-Sequence)  Freq=50  Vinit=[0, 0]  Iinit=[0, 0]  Ts=0
  Scope : Scope  NumInputPorts=4
  Scope1 : Scope
  Step : Step  Time=12+11*t_l  After=8200  SampleTime=0
  Universal Bridge : spsUniversalBridgeLib/Universal Bridge  Arms=3  SnubberResistance=1e5  SnubberCapacitance=inf  Device=Average-model based VSC  Ron=1e-3  Lon=0  ForwardVoltages="[  0  0  ]"  ForwardVoltage=0  GTOparameters=[ 10e-6 , 20e-6 ]  IGBTparameters=[ 1e-6 , 2e-6 ]  Measurements=None  Measurements_2=None  converterType=Rectifier
  Vdc : spsDCVoltageSourceLib/DC Voltage Source  Amplitude=1800  Measurements=None
  Voltage Measurement1 : spsVoltageMeasurementLib/Voltage Measurement  PhasorSimulation=off  OutputType=Complex  PSBequivalent=0
  Connection Port : PMIOPort  Side=Left
  Connection Port1 : PMIOPort  Port=2  Side=Left
  Connection Port2 : PMIOPort  Port=3  Side=Left
  Out1 : Outport
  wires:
  [Vabc_B1_13] -> Scope/3  "Inverter Voltage"
  [Iabc_B1_13] -> Scope/4  "Inverter Current"
  Voltage Measurement1/1 -> Scope1/1
  [Iabc_B3_13] -> Power (Positive-Sequence)/2, Scope/2  "PCC Current"
  Inverter Control/1(Pulses) -> Universal Bridge/1
  [Vabc_B3_13] -> Inverter Control/1(Vabc_B3)
  [Iabc_B3_13] -> Inverter Control/2(Iabc_B3)
  [Vabc_B3_13] -> Scope/1, Power (Positive-Sequence)/1  "PCC Voltage"
  Power (Positive-Sequence)/1 -> Gain2/1
  Gain2/1 -> Out1/1
  Constant1/1 -> Inverter Control/4(Iqref)
  Step/1 -> Inverter Control/3(Idref)
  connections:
  Universal Bridge/RConn1 -- Vdc/RConn1
  Universal Bridge/RConn2 -- Vdc/LConn1
  B1/LConn2 -- Voltage Measurement1/LConn2 -- Universal Bridge/LConn2
  Universal Bridge/LConn1 -- Voltage Measurement1/LConn1 -- B1/LConn1
  B3/LConn3 -- LCL Filter/RConn3
  B3/RConn3 -- B4/LConn3
  B3/RConn1 -- B4/LConn1
  Connection Port2/RConn1 -- B4/RConn3
  B3/LConn2 -- LCL Filter/RConn2
  Universal Bridge/LConn3 -- B1/LConn3
  B3/RConn2 -- B4/LConn2
  B3/LConn1 -- LCL Filter/RConn1
  B1/RConn1 -- LCL Filter/LConn1
  B1/RConn2 -- LCL Filter/LConn2
  B1/RConn3 -- LCL Filter/LConn3
  B4/RConn1 -- Connection Port/RConn1
  B4/RConn2 -- Connection Port1/RConn1

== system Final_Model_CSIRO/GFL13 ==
  B1 : spsThreePhaseVIMeasurementLib/Three-Phase V-I Measurement  VoltageMeasurement=phase-to-ground  SetLabelV=on  LabelV=Vabc_B1_14  Vpu=off  VpuLL=off  CurrentMeasurement=yes  SetLabelI=on  LabelI=Iabc_B1_14  Ipu=off  Pbase=100e6  Vbase=500e3  OutputType=Complex  PhasorSimulation=off  PSBequivalent=0
  B3 : spsThreePhaseVIMeasurementLib/Three-Phase V-I Measurement  VoltageMeasurement=phase-to-ground  SetLabelV=on  LabelV=Vabc_B3_14  Vpu=off  VpuLL=off  CurrentMeasurement=yes  SetLabelI=on  LabelI=Iabc_B3_14  Ipu=off  Pbase=100e6  Vbase=500e3  OutputType=Complex  PhasorSimulation=off  PSBequivalent=0
  B4 : spsThreePhaseVIMeasurementLib/Three-Phase V-I Measurement  VoltageMeasurement=phase-to-ground  SetLabelV=on  LabelV=Vabc_B4_14  Vpu=off  VpuLL=off  CurrentMeasurement=yes  SetLabelI=on  LabelI=Iabc_B4_14  Ipu=off  Pbase=100e6  Vbase=500e3  OutputType=Complex  PhasorSimulation=off  PSBequivalent=0
  Constant1 : Constant  Value=0  SampleTime=-1
  Gain2 : Gain  Gain=1e-8
  Inverter Control : Subsystem
  LCL Filter : Subsystem
  Power (Positive-Sequence) : spsPowerPositiveSequenceLib/Power (Positive-Sequence)  Freq=50  Vinit=[0, 0]  Iinit=[0, 0]  Ts=0
  Scope : Scope  NumInputPorts=4
  Scope1 : Scope
  Step : Step  Time=12+12*t_l  After=8200  SampleTime=0
  Universal Bridge : spsUniversalBridgeLib/Universal Bridge  Arms=3  SnubberResistance=1e5  SnubberCapacitance=inf  Device=Average-model based VSC  Ron=1e-3  Lon=0  ForwardVoltages="[  0  0  ]"  ForwardVoltage=0  GTOparameters=[ 10e-6 , 20e-6 ]  IGBTparameters=[ 1e-6 , 2e-6 ]  Measurements=None  Measurements_2=None  converterType=Rectifier
  Vdc : spsDCVoltageSourceLib/DC Voltage Source  Amplitude=1800  Measurements=None
  Voltage Measurement1 : spsVoltageMeasurementLib/Voltage Measurement  PhasorSimulation=off  OutputType=Complex  PSBequivalent=0
  Connection Port : PMIOPort  Side=Left
  Connection Port1 : PMIOPort  Port=2  Side=Left
  Connection Port2 : PMIOPort  Port=3  Side=Left
  Out1 : Outport
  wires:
  [Vabc_B1_14] -> Scope/3  "Inverter Voltage"
  [Iabc_B1_14] -> Scope/4  "Inverter Current"
  Voltage Measurement1/1 -> Scope1/1
  [Iabc_B3_14] -> Power (Positive-Sequence)/2, Scope/2  "PCC Current"
  Inverter Control/1(Pulses) -> Universal Bridge/1
  [Vabc_B3_14] -> Inverter Control/1(Vabc_B3)
  [Iabc_B3_14] -> Inverter Control/2(Iabc_B3)
  [Vabc_B3_14] -> Scope/1, Power (Positive-Sequence)/1  "PCC Voltage"
  Power (Positive-Sequence)/1 -> Gain2/1
  Gain2/1 -> Out1/1
  Constant1/1 -> Inverter Control/4(Iqref)
  Step/1 -> Inverter Control/3(Idref)
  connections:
  Universal Bridge/RConn1 -- Vdc/RConn1
  Universal Bridge/RConn2 -- Vdc/LConn1
  B1/LConn2 -- Voltage Measurement1/LConn2 -- Universal Bridge/LConn2
  Universal Bridge/LConn1 -- Voltage Measurement1/LConn1 -- B1/LConn1
  B3/LConn3 -- LCL Filter/RConn3
  B3/RConn3 -- B4/LConn3
  B3/RConn1 -- B4/LConn1
  Connection Port2/RConn1 -- B4/RConn3
  B3/LConn2 -- LCL Filter/RConn2
  Universal Bridge/LConn3 -- B1/LConn3
  B3/RConn2 -- B4/LConn2
  B3/LConn1 -- LCL Filter/RConn1
  B1/RConn1 -- LCL Filter/LConn1
  B1/RConn2 -- LCL Filter/LConn2
  B1/RConn3 -- LCL Filter/LConn3
  B4/RConn1 -- Connection Port/RConn1
  B4/RConn2 -- Connection Port1/RConn1

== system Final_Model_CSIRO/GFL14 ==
  B1 : spsThreePhaseVIMeasurementLib/Three-Phase V-I Measurement  VoltageMeasurement=phase-to-ground  SetLabelV=on  LabelV=Vabc_B1_15  Vpu=off  VpuLL=off  CurrentMeasurement=yes  SetLabelI=on  LabelI=Iabc_B1_15  Ipu=off  Pbase=100e6  Vbase=500e3  OutputType=Complex  PhasorSimulation=off  PSBequivalent=0
  B3 : spsThreePhaseVIMeasurementLib/Three-Phase V-I Measurement  VoltageMeasurement=phase-to-ground  SetLabelV=on  LabelV=Vabc_B3_15  Vpu=off  VpuLL=off  CurrentMeasurement=yes  SetLabelI=on  LabelI=Iabc_B3_15  Ipu=off  Pbase=100e6  Vbase=500e3  OutputType=Complex  PhasorSimulation=off  PSBequivalent=0
  B4 : spsThreePhaseVIMeasurementLib/Three-Phase V-I Measurement  VoltageMeasurement=phase-to-ground  SetLabelV=on  LabelV=Vabc_B4_15  Vpu=off  VpuLL=off  CurrentMeasurement=yes  SetLabelI=on  LabelI=Iabc_B4_15  Ipu=off  Pbase=100e6  Vbase=500e3  OutputType=Complex  PhasorSimulation=off  PSBequivalent=0
  Constant1 : Constant  Value=0  SampleTime=-1
  Gain2 : Gain  Gain=1e-8
  Inverter Control : Subsystem
  LCL Filter : Subsystem
  Power (Positive-Sequence) : spsPowerPositiveSequenceLib/Power (Positive-Sequence)  Freq=50  Vinit=[0, 0]  Iinit=[0, 0]  Ts=0
  Scope : Scope  NumInputPorts=4
  Scope1 : Scope
  Step : Step  Time=10+13*t_l  After=8200  SampleTime=0
  Universal Bridge : spsUniversalBridgeLib/Universal Bridge  Arms=3  SnubberResistance=1e5  SnubberCapacitance=inf  Device=Average-model based VSC  Ron=1e-3  Lon=0  ForwardVoltages="[  0  0  ]"  ForwardVoltage=0  GTOparameters=[ 10e-6 , 20e-6 ]  IGBTparameters=[ 1e-6 , 2e-6 ]  Measurements=None  Measurements_2=None  converterType=Rectifier
  Vdc : spsDCVoltageSourceLib/DC Voltage Source  Amplitude=1800  Measurements=None
  Voltage Measurement1 : spsVoltageMeasurementLib/Voltage Measurement  PhasorSimulation=off  OutputType=Complex  PSBequivalent=0
  Connection Port : PMIOPort  Side=Left
  Connection Port1 : PMIOPort  Port=2  Side=Left
  Connection Port2 : PMIOPort  Port=3  Side=Left
  Out1 : Outport
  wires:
  [Vabc_B1_15] -> Scope/3  "Inverter Voltage"
  [Iabc_B1_15] -> Scope/4  "Inverter Current"
  Voltage Measurement1/1 -> Scope1/1
  [Iabc_B3_15] -> Power (Positive-Sequence)/2, Scope/2  "PCC Current"
  Inverter Control/1(Pulses) -> Universal Bridge/1
  [Vabc_B3_15] -> Inverter Control/1(Vabc_B3)
  [Iabc_B3_15] -> Inverter Control/2(Iabc_B3)
  [Vabc_B3_15] -> Scope/1, Power (Positive-Sequence)/1  "PCC Voltage"
  Power (Positive-Sequence)/1 -> Gain2/1
  Gain2/1 -> Out1/1
  Constant1/1 -> Inverter Control/4(Iqref)
  Step/1 -> Inverter Control/3(Idref)
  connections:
  Universal Bridge/RConn1 -- Vdc/RConn1
  Universal Bridge/RConn2 -- Vdc/LConn1
  B1/LConn2 -- Voltage Measurement1/LConn2 -- Universal Bridge/LConn2
  Universal Bridge/LConn1 -- Voltage Measurement1/LConn1 -- B1/LConn1
  B3/LConn3 -- LCL Filter/RConn3
  B3/RConn3 -- B4/LConn3
  B3/RConn1 -- B4/LConn1
  Connection Port2/RConn1 -- B4/RConn3
  B3/LConn2 -- LCL Filter/RConn2
  Universal Bridge/LConn3 -- B1/LConn3
  B3/RConn2 -- B4/LConn2
  B3/LConn1 -- LCL Filter/RConn1
  B1/RConn1 -- LCL Filter/LConn1
  B1/RConn2 -- LCL Filter/LConn2
  B1/RConn3 -- LCL Filter/LConn3
  B4/RConn1 -- Connection Port/RConn1
  B4/RConn2 -- Connection Port1/RConn1

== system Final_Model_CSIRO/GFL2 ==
  B1 : spsThreePhaseVIMeasurementLib/Three-Phase V-I Measurement  VoltageMeasurement=phase-to-ground  SetLabelV=on  LabelV=Vabc_B1_3  Vpu=off  VpuLL=off  CurrentMeasurement=yes  SetLabelI=on  LabelI=Iabc_B1_3  Ipu=off  Pbase=100e6  Vbase=500e3  OutputType=Complex  PhasorSimulation=off  PSBequivalent=0
  B3 : spsThreePhaseVIMeasurementLib/Three-Phase V-I Measurement  VoltageMeasurement=phase-to-ground  SetLabelV=on  LabelV=Vabc_B3_3  Vpu=off  VpuLL=off  CurrentMeasurement=yes  SetLabelI=on  LabelI=Iabc_B3_3  Ipu=off  Pbase=100e6  Vbase=500e3  OutputType=Complex  PhasorSimulation=off  PSBequivalent=0
  B4 : spsThreePhaseVIMeasurementLib/Three-Phase V-I Measurement  VoltageMeasurement=phase-to-ground  SetLabelV=on  LabelV=Vabc_B4_3  Vpu=off  VpuLL=off  CurrentMeasurement=yes  SetLabelI=on  LabelI=Iabc_B4_3  Ipu=off  Pbase=100e6  Vbase=500e3  OutputType=Complex  PhasorSimulation=off  PSBequivalent=0
  Constant1 : Constant  Value=0  SampleTime=-1
  Gain2 : Gain  Gain=1e-8
  Inverter Control : Subsystem
  LCL Filter : Subsystem
  Power (Positive-Sequence) : spsPowerPositiveSequenceLib/Power (Positive-Sequence)  Freq=50  Vinit=[0, 0]  Iinit=[0, 0]  Ts=0
  Scope : Scope  NumInputPorts=4
  Scope1 : Scope
  Step : Step  Time=12+t_l  After=8200  SampleTime=0
  Universal Bridge : spsUniversalBridgeLib/Universal Bridge  Arms=3  SnubberResistance=1e5  SnubberCapacitance=inf  Device=Average-model based VSC  Ron=1e-3  Lon=0  ForwardVoltages="[  0  0  ]"  ForwardVoltage=0  GTOparameters=[ 10e-6 , 20e-6 ]  IGBTparameters=[ 1e-6 , 2e-6 ]  Measurements=None  Measurements_2=None  converterType=Rectifier
  Vdc : spsDCVoltageSourceLib/DC Voltage Source  Amplitude=1800  Measurements=None
  Voltage Measurement1 : spsVoltageMeasurementLib/Voltage Measurement  PhasorSimulation=off  OutputType=Complex  PSBequivalent=0
  Connection Port : PMIOPort  Side=Left
  Connection Port1 : PMIOPort  Port=2  Side=Left
  Connection Port2 : PMIOPort  Port=3  Side=Left
  Out1 : Outport
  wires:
  [Vabc_B1_3] -> Scope/3  "Inverter Voltage"
  [Iabc_B1_3] -> Scope/4  "Inverter Current"
  Voltage Measurement1/1 -> Scope1/1
  [Iabc_B3_3] -> Power (Positive-Sequence)/2, Scope/2  "PCC Current"
  Inverter Control/1(Pulses) -> Universal Bridge/1
  [Vabc_B3_3] -> Inverter Control/1(Vabc_B3)
  [Iabc_B3_3] -> Inverter Control/2(Iabc_B3)
  [Vabc_B3_3] -> Scope/1, Power (Positive-Sequence)/1  "PCC Voltage"
  Power (Positive-Sequence)/1 -> Gain2/1
  Gain2/1 -> Out1/1
  Constant1/1 -> Inverter Control/4(Iqref)
  Step/1 -> Inverter Control/3(Idref)
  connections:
  Universal Bridge/RConn1 -- Vdc/RConn1
  Universal Bridge/RConn2 -- Vdc/LConn1
  B1/LConn2 -- Voltage Measurement1/LConn2 -- Universal Bridge/LConn2
  Universal Bridge/LConn1 -- Voltage Measurement1/LConn1 -- B1/LConn1
  B3/LConn3 -- LCL Filter/RConn3
  B3/RConn3 -- B4/LConn3
  B3/RConn1 -- B4/LConn1
  Connection Port2/RConn1 -- B4/RConn3
  B3/LConn2 -- LCL Filter/RConn2
  Universal Bridge/LConn3 -- B1/LConn3
  B3/RConn2 -- B4/LConn2
  B3/LConn1 -- LCL Filter/RConn1
  B1/RConn1 -- LCL Filter/LConn1
  B1/RConn2 -- LCL Filter/LConn2
  B1/RConn3 -- LCL Filter/LConn3
  B4/RConn1 -- Connection Port/RConn1
  B4/RConn2 -- Connection Port1/RConn1

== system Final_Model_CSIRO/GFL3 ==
  B1 : spsThreePhaseVIMeasurementLib/Three-Phase V-I Measurement  VoltageMeasurement=phase-to-ground  SetLabelV=on  LabelV=Vabc_B1_4  Vpu=off  VpuLL=off  CurrentMeasurement=yes  SetLabelI=on  LabelI=Iabc_B1_4  Ipu=off  Pbase=100e6  Vbase=500e3  OutputType=Complex  PhasorSimulation=off  PSBequivalent=0
  B3 : spsThreePhaseVIMeasurementLib/Three-Phase V-I Measurement  VoltageMeasurement=phase-to-ground  SetLabelV=on  LabelV=Vabc_B3_4  Vpu=off  VpuLL=off  CurrentMeasurement=yes  SetLabelI=on  LabelI=Iabc_B3_4  Ipu=off  Pbase=100e6  Vbase=500e3  OutputType=Complex  PhasorSimulation=off  PSBequivalent=0
  B4 : spsThreePhaseVIMeasurementLib/Three-Phase V-I Measurement  VoltageMeasurement=phase-to-ground  SetLabelV=on  LabelV=Vabc_B4_4  Vpu=off  VpuLL=off  CurrentMeasurement=yes  SetLabelI=on  LabelI=Iabc_B4_4  Ipu=off  Pbase=100e6  Vbase=500e3  OutputType=Complex  PhasorSimulation=off  PSBequivalent=0
  Constant1 : Constant  Value=0  SampleTime=-1
  Gain2 : Gain  Gain=1e-8
  Inverter Control : Subsystem
  LCL Filter : Subsystem
  Power (Positive-Sequence) : spsPowerPositiveSequenceLib/Power (Positive-Sequence)  Freq=50  Vinit=[0, 0]  Iinit=[0, 0]  Ts=0
  Scope : Scope  NumInputPorts=4
  Scope1 : Scope
  Step : Step  Time=12+2*t_l  After=8200  SampleTime=0
  Universal Bridge : spsUniversalBridgeLib/Universal Bridge  Arms=3  SnubberResistance=1e5  SnubberCapacitance=inf  Device=Average-model based VSC  Ron=1e-3  Lon=0  ForwardVoltages="[  0  0  ]"  ForwardVoltage=0  GTOparameters=[ 10e-6 , 20e-6 ]  IGBTparameters=[ 1e-6 , 2e-6 ]  Measurements=None  Measurements_2=None  converterType=Rectifier
  Vdc : spsDCVoltageSourceLib/DC Voltage Source  Amplitude=1800  Measurements=None
  Voltage Measurement1 : spsVoltageMeasurementLib/Voltage Measurement  PhasorSimulation=off  OutputType=Complex  PSBequivalent=0
  Connection Port : PMIOPort  Side=Left
  Connection Port1 : PMIOPort  Port=2  Side=Left
  Connection Port2 : PMIOPort  Port=3  Side=Left
  Out1 : Outport
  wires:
  [Vabc_B1_4] -> Scope/3  "Inverter Voltage"
  [Iabc_B1_4] -> Scope/4  "Inverter Current"
  Voltage Measurement1/1 -> Scope1/1
  [Iabc_B3_4] -> Power (Positive-Sequence)/2, Scope/2  "PCC Current"
  Inverter Control/1(Pulses) -> Universal Bridge/1
  [Vabc_B3_4] -> Inverter Control/1(Vabc_B3)
  [Iabc_B3_4] -> Inverter Control/2(Iabc_B3)
  [Vabc_B3_4] -> Scope/1, Power (Positive-Sequence)/1  "PCC Voltage"
  Power (Positive-Sequence)/1 -> Gain2/1
  Gain2/1 -> Out1/1
  Constant1/1 -> Inverter Control/4(Iqref)
  Step/1 -> Inverter Control/3(Idref)
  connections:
  Universal Bridge/RConn1 -- Vdc/RConn1
  Universal Bridge/RConn2 -- Vdc/LConn1
  B1/LConn2 -- Voltage Measurement1/LConn2 -- Universal Bridge/LConn2
  Universal Bridge/LConn1 -- Voltage Measurement1/LConn1 -- B1/LConn1
  B3/LConn3 -- LCL Filter/RConn3
  B3/RConn3 -- B4/LConn3
  B3/RConn1 -- B4/LConn1
  Connection Port2/RConn1 -- B4/RConn3
  B3/LConn2 -- LCL Filter/RConn2
  Universal Bridge/LConn3 -- B1/LConn3
  B3/RConn2 -- B4/LConn2
  B3/LConn1 -- LCL Filter/RConn1
  B1/RConn1 -- LCL Filter/LConn1
  B1/RConn2 -- LCL Filter/LConn2
  B1/RConn3 -- LCL Filter/LConn3
  B4/RConn1 -- Connection Port/RConn1
  B4/RConn2 -- Connection Port1/RConn1
